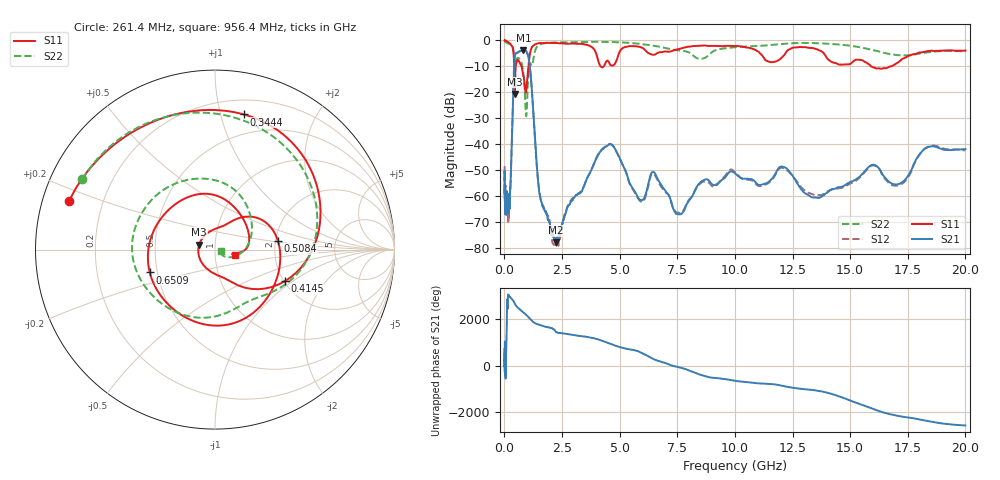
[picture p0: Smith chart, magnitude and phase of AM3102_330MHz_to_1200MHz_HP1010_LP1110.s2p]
! Date/Time: Tue, Sep 11, 2018 5:19 PM
! Network Analyzer: Agilent Technologies E8362B Rev: A.07.50.63
! Sweep from 0.010 to 20.000 GHz, 1601 Points, Sweep Type: LOG
! Power Supply: 4.949 V, 0.001 A
# Hz S DB R 50
!freq MagS11 AngS11 MagS21 AngS21 MagS12 AngS12 MagS22 AngS22
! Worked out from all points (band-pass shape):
!   1601 points, 10 MHz to 20 GHz, reference 50 ohm
!   highest |S21| = -3.64 dB at 821.5 MHz (marker M1); lowest = -77.9 dB at 2.238 GHz (marker M2)
!   |S21| within 3 dB of the highest: 445.6 MHz to 1.047 GHz (601.1 MHz wide, 80.6 % of centre)
!   lowest |S11| = -20.7 dB at 451.5 MHz (marker M3), VSWR 1.20, Z = 41.8 + j2.38 ohm
!   |S11| at or under -10 dB: 743.5 MHz to 1.042 GHz (299 MHz wide, 33.5 % of centre); 4.174 GHz to 4.312 GHz (138.6 MHz wide, 3.27 % of centre); 15.91 GHz to 16.76 GHz (851.2 MHz wide, 5.21 % of centre)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
!   |S22| runs from -29.2 to -0.2 dB; largest |S21 - S12| = 0.0091
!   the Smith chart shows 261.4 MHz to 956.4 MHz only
!   S11 on the Smith chart (normalised r, x): 261.4 MHz: 0.08, +0.16; 344.4 MHz: 0.32, +1.19; 414.5 MHz: 2.02, -0.87; 508.4 MHz: 2.06, +0.23; 650.9 MHz: 0.45, -0.14; 956.4 MHz: 1.25, -0.07
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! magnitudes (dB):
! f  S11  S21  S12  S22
! 10 MHz  0.0  -53.9  -48.9  -0.2
! 35.55 MHz  0.0  -64.6  -62.9  -0.5
! 126.4 MHz  -0.4  -66.5  -64.0  -1.0
! 261.4 MHz  -1.4  -56.5  -56.7  -1.5
! 344.4 MHz  -2.3  -32.2  -32.2  -2.5
! 414.5 MHz  -7.4  -11.4  -11.4  -5.9
! 447.2 MHz  -20.5  -6.5  -6.6  -9.0
! 451.5 MHz  -20.7  -6.2  -6.3  -9.2
! 508.4 MHz  -9.0  -4.9  -5.0  -7.9
! 650.9 MHz  -8.3  -4.2  -4.3  -7.0
! 821.5 MHz  -13.6  -3.6  -3.7  -12.4
! 956.4 MHz  -18.7  -4.2  -4.3  -28.8
! 1.14 GHz  -3.9  -13.3  -13.4  -9.0
! 1.59 GHz  -1.0  -62.0  -61.8  -1.4
! 2.238 GHz  -0.9  -77.9  -78.2  -0.8
! 4.436 GHz  -7.9  -40.8  -40.7  -0.5
! 5.652 GHz  -2.2  -58.2  -58.6  -1.1
! 6.549 GHz  -5.4  -51.5  -52.2  -2.1
! 7.588 GHz  -3.3  -67.1  -66.5  -3.9
! 12.09 GHz  -6.1  -48.7  -49.2  -1.3
! 13.55 GHz  -3.3  -60.7  -59.8  -1.1
! 20 GHz  -3.9  -41.9  -42.4  -4.2
